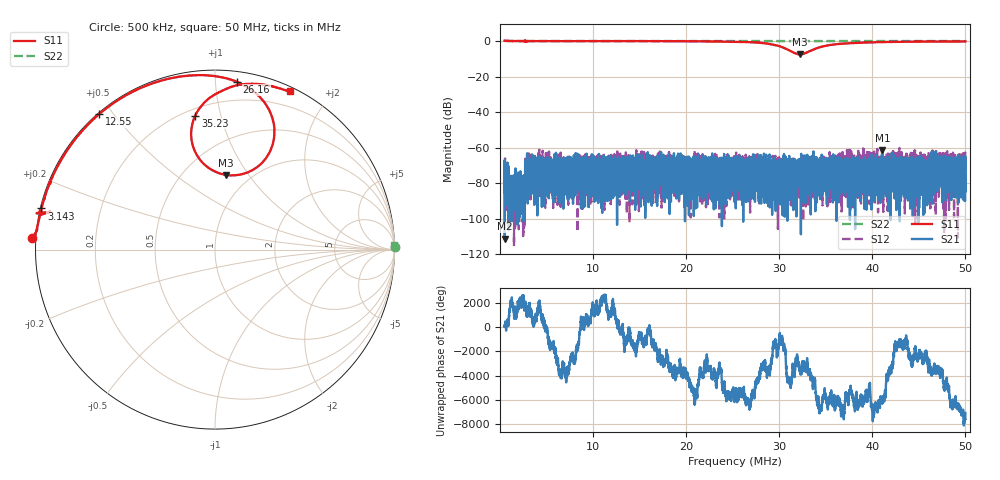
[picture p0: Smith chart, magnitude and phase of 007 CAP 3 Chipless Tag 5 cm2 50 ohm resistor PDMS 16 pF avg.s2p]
!  26/06/2025  15:33:34
! Ref Plane: 0.000 mm
# MHZ S MA R  50
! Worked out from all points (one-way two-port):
!   10001 points, 500 kHz to 50 MHz, reference 50 ohm
!   highest |S21| = -61.34 dB at 41.09 MHz (marker M1); lowest = -111.2 dB at 519.8 kHz (marker M2)
!   lowest |S11| = -7.5 dB at 32.22 MHz (marker M3), VSWR 2.45, Z = 39.2 + j39.6 ohm
!   |S11| at or under -10 dB: nowhere
!   |S22| runs from -0.3 to 0.3 dB; largest |S21 - S12| = 0.0012
!   S11 on the Smith chart (normalised r, x): 500 kHz: -0.01, +0.03; 3.143 MHz: 0.00, +0.12; 12.55 MHz: 0.00, +0.46; 26.16 MHz: 0.07, +1.14; 35.23 MHz: 0.24, +0.83; 50 MHz: 0.04, +1.58
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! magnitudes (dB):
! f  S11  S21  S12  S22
! 500 kHz  0.2  -85.3  -73.8  0.0
! 519.8 kHz  0.2  -111.2  -72.1  0.0
! 752.5 kHz  0.1  -71.1  -86.4  0.0
! 1.149 MHz  0.0  -78.0  -91.2  0.0
! 2.455 MHz  0.0  -78.4  -90.0  0.0
! 3.143 MHz  -0.1  -73.6  -75.6  0.0
! 6.91 MHz  -0.1  -86.3  -81.2  0.0
! 8.752 MHz  -0.1  -82.6  -85.1  0.0
! 12.55 MHz  -0.1  -75.7  -70.5  0.0
! 17 MHz  -0.1  -72.7  -64.5  0.0
! 24.84 MHz  -0.3  -76.9  -77.7  0.0
! 25.25 MHz  -0.4  -74.4  -77.6  0.0
! 26.16 MHz  -0.5  -79.5  -73.8  0.0
! 29.47 MHz  -2.1  -65.5  -74.4  0.0
! 32.22 MHz  -7.5  -79.4  -76.6  0.0
! 33.5 MHz  -5.1  -77.5  -67.8  0.0
! 35.23 MHz  -2.4  -68.6  -70.4  0.0
! 41.09 MHz  -0.6  -61.3  -71.2  0.0
! 41.75 MHz  -0.5  -72.2  -80.6  0.0
! 48.6 MHz  -0.3  -75.1  -71.1  0.0
! 49.75 MHz  -0.2  -77.4  -63.2  0.0
! 50 MHz  -0.2  -79.9  -67.4  0.0
